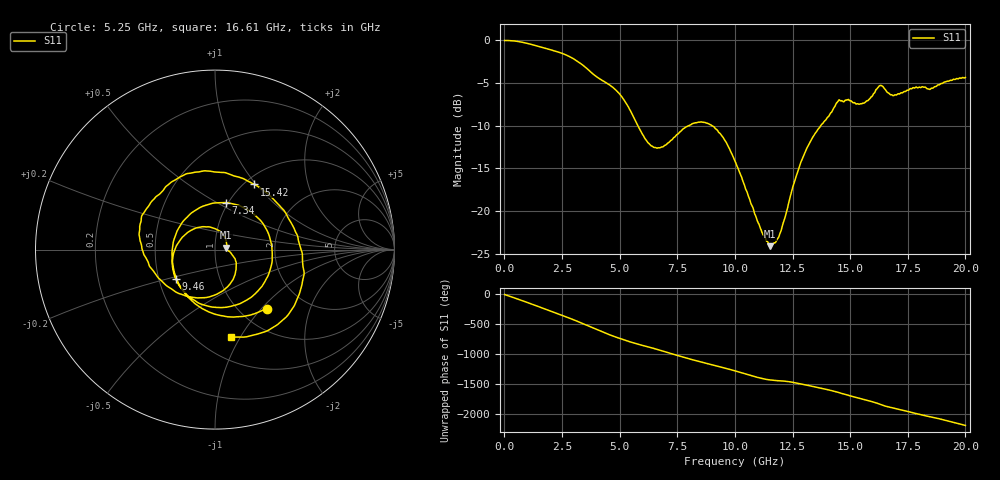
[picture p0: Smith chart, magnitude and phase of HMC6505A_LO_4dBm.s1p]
! Analog Devices, Inc.
! 1 Analog Way
! Wilmington, MA 01887
! http://www.analog.com
! Date:  2021-09-17 NN
! Board Name:  EV1HMC6505ALC5 (125487-1) with HMC6505ALC5 installed
! File Description:  S-Parameters for evaluation board without connectors or board loss de-embedded
! File Generation:  Calibrated Network Analyzer
! Chip Part Number:  HMC6505A
! Chip Description:  GaAs, MMIC, IQ Upconverter
! Chip Frequency:  5.5 to 8.6 GHz
! Chip Package:  LCC, 4.9 x 4.9 x 1 mm
! Chip State:
!  Temperature:  25C
!  LO Power:  4dBm
! Note:
!  Analog Devices supplies this data as a sample of measured data at the evaluation board
!  ports for this product.  Your particular data for this product may vary.
!  Analog Devices reserves the right to change this data at anytime.
!  All lines below in this file are as is from the Network Analyzer.
!Keysight Technologies,N5245A,MY49151104,A.10.65.16
!Date: Wednesday, September 15, 2021 13:45:08
!Correction: S11(Full 2 Port(1,2))
!S1P File: Measurement: S11:
# Hz S  dB  R 50
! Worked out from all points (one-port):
!   2000 points, 10 MHz to 20 GHz, reference 50 ohm
!   lowest |S11| = -24.1 dB at 11.51 GHz (marker M1), VSWR 1.13, Z = 56.5 + j1.13 ohm
!   |S11| at or under -10 dB: 5.794 GHz to 7.979 GHz (2.185 GHz wide, 31.7 % of centre); 9.01 GHz to 13.72 GHz (4.706 GHz wide, 41.4 % of centre)
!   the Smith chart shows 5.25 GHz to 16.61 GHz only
!   S11 on the Smith chart (normalised r, x): 5.25 GHz: 1.31, -1.07; 7.34 GHz: 0.98, +0.55; 9.46 GHz: 0.61, -0.22; 15.42 GHz: 1.10, +0.98; 16.61 GHz: 0.71, -0.92
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1e7  -0.01 -1.4
6.7e8  -0.16 -89.4
1.29e9  -0.55 -176.0
1.9e9  -1.02 96.5
2.51e9  -1.53 9.1
3.1e9  -2.32 -79.3
3.66e9  -3.48 -170.5
4.25e9  -4.71 92.8
5.01e9  -6.31 -17.7
5.25e9  -7.20 -48.9
6.2e9  -11.87 -154.7
7.34e9  -11.40 77.0
7.51e9  -10.99 57.4
8.69e9  -9.60 -66.9
9.46e9  -11.26 -143.1
1.001e10  -14.17 160.2
1.151e10  -24.10 9.2
1.251e10  -17.18 -31.2
1.371e10  -10.03 -128.7
1.445e10  -7.21 164.1
1.501e10  -7.09 100.6
1.542e10  -7.46 59.0
1.611e10  -5.79 -14.8
1.661e10  -6.08 -79.6
1.751e10  -5.84 -161.1
1.884e10  -5.20 79.9
1.949e10  -4.55 17.8
2e10  -4.33 -34.4
